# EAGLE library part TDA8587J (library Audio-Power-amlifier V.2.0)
4 ´ 25 W BTL power amplifier and multiple voltage regulator with power switch
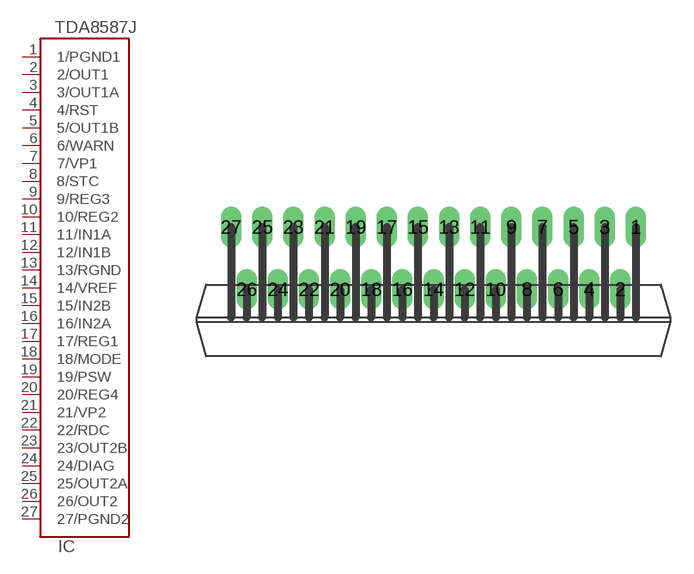
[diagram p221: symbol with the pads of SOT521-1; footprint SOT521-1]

Designator prefix IC

## TDA8587J  [SOT521-1]
1  1/PGND1  pwr
2  2/OUT1  out
3  3/OUT1A  out
4  4/RST  out
5  5/OUT1B  out
6  6/WARN  out
7  7/VP1  pwr
8  8/STC
9  9/REG3  out
10  10/REG2  out
11  11/IN1A  in
12  12/IN1B  in
13  13/RGND  pwr
14  14/VREF
15  15/IN2B  in
16  16/IN2A  in
17  17/REG1  out
18  18/MODE  in
19  19/PSW  out
20  20/REG4  out
21  21/VP2  pwr
22  22/RDC
23  23/OUT2B  out
24  24/DIAG  out
25  25/OUT2A  out
26  26/OUT2  out
27  27/PGND2  pwr

## Footprint SOT521-1 (pad centres in mm)
drill 0.8 long: 1 13,4; 2 12,0; 3 11,4; 4 10,0; 5 9,4; 6 8,0; 7 7,4; 8 6,0; 9 5,4; 10 4,0; 11 3,4; 12 2,0; 13 1,4; 14 0,0; 15 -1,4; 16 -2,0; 17 -3,4; 18 -4,0; 19 -5,4; 20 -6,0; 21 -7,4; 22 -8,0; 23 -9,4; 24 -10,0; 25 -11,4; 26 -12,0; 27 -13,4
